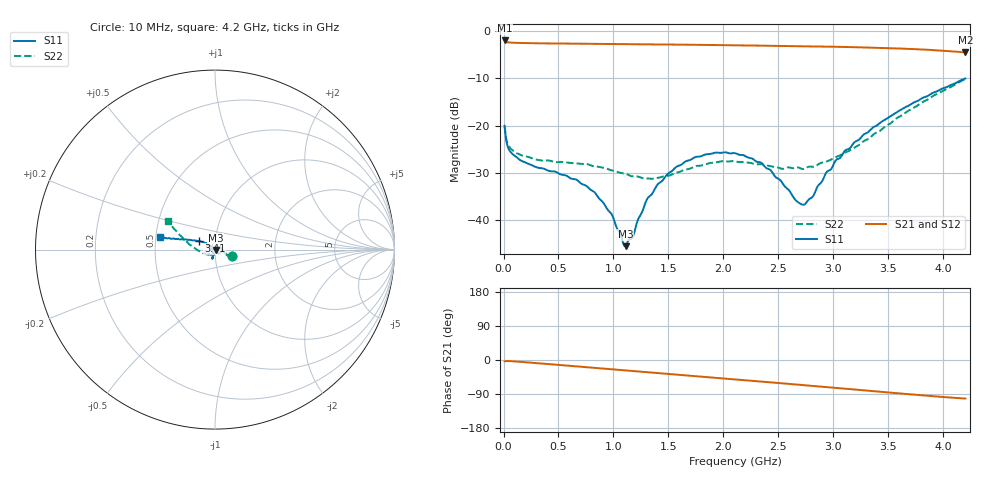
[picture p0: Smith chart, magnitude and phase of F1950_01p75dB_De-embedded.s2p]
! Integrated Device Technology
! Corporate Headquarters
! 6024 Silver Creek Valley Road
! San Jose, CA 95138  USA
! Phone:  1-408-284-8200
! Toll Free:  1-800-223-1366
! Webpage:  http://www.idt.com/
! Timing and RF Division
! 515 Groton Road, Suite 102
! Westford, MA 01886-6024
! Device:  F1950
! Description: 7-bit 0.25 dB Digital Step Attenuator
! Frequency:  150.0 -  4000.00 MHz
! Package:  4x4 mm Thin QFN Plastic Package: 24 pin
! Ports:  2 RF, 12 DC
!  Pin  1  = D0
!  Pin  2  = VDD
!  Pin  3  = Vmode
!  Pin  4  = GND
!  Pin  5  = RF1  =  Port 1
!  Pin  6  = GND
!  Pin  7  = GND
!  Pin  8  = GND
!  Pin  9  = GND
!  Pin 10  = GND
!  Pin 11  = GND
!  Pin 12  = GND
!  Pin 13  = GND
!  Pin 14  = RF2  =  Port 2
!  Pin 15  = GND
!  Pin 16  = LE
!  Pin 17  = CLK
!  Pin 18  = DATE
!  Pin 19  = D6
!  Pin 20  = D5
!  Pin 21  = D4
!  Pin 22  = D3
!  Pin 23  = D2
!  Pin 24  = D1
! State:  7
! Atten State:  1.75 dB
! Voltage:  +5.00 Volts
! Current:  Not Measured mA
! Data:  The device was measured on a the F195X evaluation board which has
!  individual transmission lines to the RF pins.  Data was collected
!  using a calibrated network analyzer.  The evaluation board was
!  de-embedded using a TRL calibration technique.
!  The reference plane is the edge of the package pin.
! Misc:  Board 2019
!  Action Tracker AT0250
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# GHz S dB R 50
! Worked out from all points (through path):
!   420 points, 10 MHz to 4.2 GHz, reference 50 ohm
!   highest |S21| = -2.02 dB at 10 MHz (marker M1); lowest = -4.5 dB at 4.2 GHz (marker M2)
!   group delay of S21, straight-line fit = 67.1 ps
!   lowest |S11| = -45.4 dB at 1.11 GHz (marker M3), VSWR 1.01, Z = 50.5 - j0.257 ohm
!   |S11| at or under -10 dB: start of sweep to end of sweep
!   |S22| runs from -31.2 to -10.2 dB; largest |S21 - S12| = 0.00091
!   S11 on the Smith chart (normalised r, x): 10 MHz: 1.20, -0.09; 3.41 GHz: 0.83, +0.08; 4.2 GHz: 0.53, +0.08
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0.01  -20.04 -22.2  -2.02 -3.3  -2.02 -3.3  -20.08 -21.4
0.06  -25.43 -16.8  -2.46 -2.9  -2.46 -2.9  -24.70 -17.2
0.15  -27.25 -7.6  -2.55 -4.7  -2.54 -4.7  -26.10 -11.3
0.71  -32.27 33.4  -2.70 -17.9  -2.70 -17.9  -28.08 -12.8
0.91  -36.33 33.8  -2.74 -22.7  -2.74 -22.7  -28.91 -23.7
0.98  -38.57 27.0  -2.76 -24.4  -2.76 -24.4  -29.41 -29.7
1.09  -44.93 -10.8  -2.78 -27.0  -2.78 -27.0  -30.06 -41.9
1.11  -45.43 -28.4  -2.78 -27.4  -2.78 -27.4  -30.15 -44.1
1.18  -43.24 -70.5  -2.80 -29.1  -2.80 -29.1  -30.64 -53.5
1.3  -35.73 -98.0  -2.82 -32.0  -2.82 -32.0  -31.13 -72.1
1.41  -32.19 -103.0  -2.85 -34.6  -2.85 -34.6  -30.97 -89.9
1.57  -28.73 -106.3  -2.89 -38.4  -2.89 -38.5  -29.91 -112.5
1.74  -26.66 -107.1  -2.93 -42.5  -2.93 -42.6  -28.58 -129.1
2.11  -25.83 -106.4  -3.04 -51.4  -3.04 -51.5  -27.58 -145.1
2.35  -27.95 -108.3  -3.12 -57.2  -3.12 -57.2  -28.14 -144.6
2.7  -36.49 -156.5  -3.22 -65.6  -3.22 -65.6  -28.99 -134.5
2.74  -36.61 -172.5  -3.24 -66.6  -3.24 -66.6  -29.04 -135.5
2.81  -35.03 165.4  -3.27 -68.3  -3.26 -68.3  -28.67 -134.7
3.03  -27.13 145.1  -3.36 -73.8  -3.36 -73.9  -26.56 -143.9
3.41  -19.69 152.6  -3.57 -83.4  -3.57 -83.4  -21.28 -173.4
3.51  -18.13 155.6  -3.64 -85.9  -3.64 -85.9  -19.66 179.3
4.2  -10.03 167.1  -4.54 -101.8  -4.53 -101.8  -10.17 148.6
